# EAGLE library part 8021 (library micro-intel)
MICROCOMPUTER/PERIPHERAL DEVICE
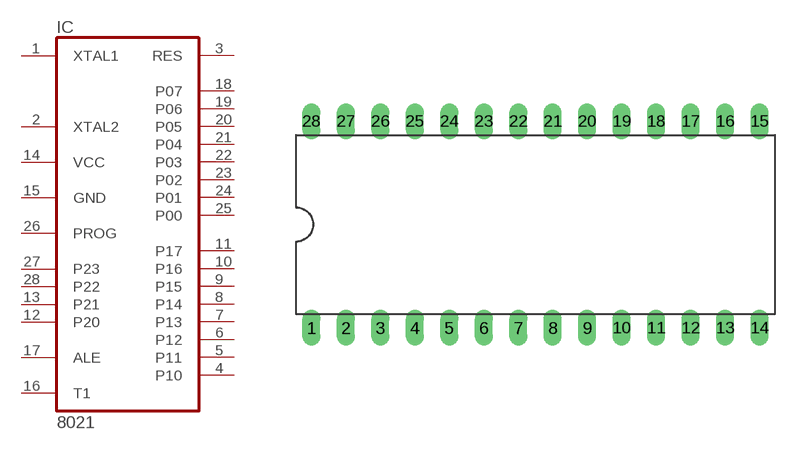
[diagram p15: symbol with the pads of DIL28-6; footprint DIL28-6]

Designator prefix IC

## 8021 (OC_FARNELL: unknown; OC_NEWARK: unknown)  [DIL28-6]
1  XTAL1  in
2  XTAL2  in
3  RES  in
4  P10
5  P11
6  P12
7  P13
8  P14
9  P15
10  P16
11  P17
12  P20
13  P21
14  VCC  pwr
15  GND  pwr
16  T1  in
17  ALE  out
18  P07
19  P06
20  P05
21  P04
22  P03
23  P02
24  P01
25  P00
26  PROG  out
27  P23
28  P22

## Footprint DIL28-6 (pad centres in mm)
Dual In Line Package 0.6 inch
drill 0.813 long: 1 -16.51,-7.62; 2 -13.97,-7.62; 3 -11.43,-7.62; 4 -8.89,-7.62; 5 -6.35,-7.62; 6 -3.81,-7.62; 7 -1.27,-7.62; 8 1.27,-7.62; 9 3.81,-7.62; 10 6.35,-7.62; 11 8.89,-7.62; 12 11.43,-7.62; 13 13.97,-7.62; 14 16.51,-7.62; 15 16.51,7.62; 16 13.97,7.62; 17 11.43,7.62; 18 8.89,7.62; 19 6.35,7.62; 20 3.81,7.62; 21 1.27,7.62; 22 -1.27,7.62; 23 -3.81,7.62; 24 -6.35,7.62; 25 -8.89,7.62; 26 -11.43,7.62; 27 -13.97,7.62; 28 -16.51,7.62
